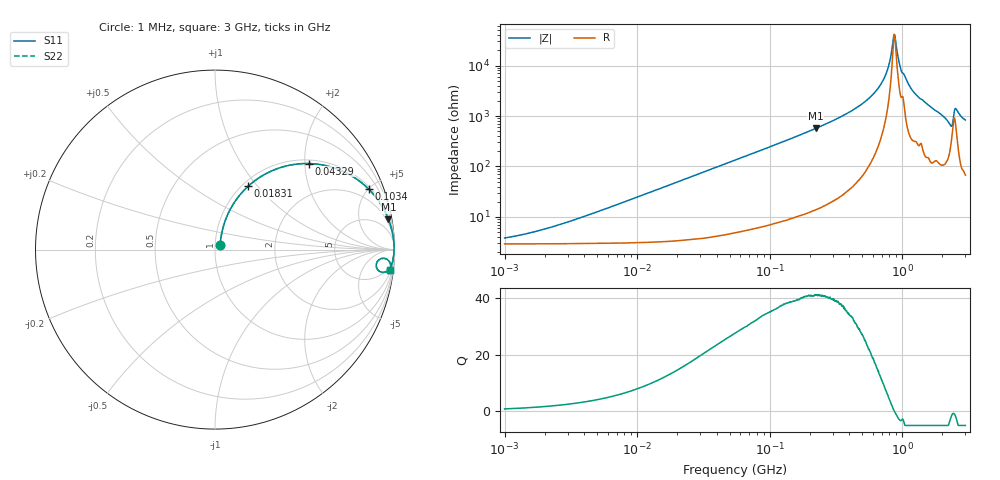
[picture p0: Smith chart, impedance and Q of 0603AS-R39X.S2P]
!s-Parameter Generated by FASTRON Sdn. Bhd.
!FASTRON P/N : 0603AS-R39X
!Keysight Technologies: E4991B_MY54100416_A.01.15
!Date: Tue Oct 17 16:06:11 2023
!Date created: Tue Oct 17 16:06:11 2023
!Version  : Rev01 Tue Oct 17 16:06:11 2023
!Data & Calibration Information:
!Freq	S11	S21	S12	S22
!PortZ  Port1:50+j0  Port2:50+j0
!When reading reference impedance value at option line is always used.
! Remarks : This data is being provided solely for informational purposes.
# Hz S dB R 50
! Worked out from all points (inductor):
!   1601 points, 1 MHz to 3 GHz, reference 50 ohm
!   read as one part in series: L = 390 nH near 3.618 MHz
!   highest Q = 41 at 222.4 MHz (marker M1), where L = 405 nH
!   self-resonance near 871.6 MHz
!   S11 on the Smith chart (normalised r, x): 1 MHz: 1.06, +0.05; 18.31 MHz: 1.07, +0.89; 43.29 MHz: 1.09, +2.11; 103.4 MHz: 1.14, +5.04; 3 GHz: 2, -17
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1000000  -28.61 38.9  -0.25 -1.4  -0.25 -1.4  -28.61 38.9
3804036  -20.47 67.2  -0.29 -5.2  -0.29 -5.2  -20.47 67.2
1.447069e7  -9.76 65.9  -0.75 -18.9  -0.75 -18.9  -9.76 65.9
1.830753e7  -8.00 62.4  -1.03 -23.4  -1.03 -23.4  -8.00 62.4
4.329325e7  -2.96 42.4  -3.42 -45.3  -3.42 -45.3  -2.96 42.4
5.477226e7  -2.09 36.1  -4.58 -51.8  -4.58 -51.8  -2.09 36.1
1.034087e8  -0.72 21.4  -8.75 -67.0  -8.75 -67.0  -0.72 21.4
2.083556e8  -0.19 10.7  -14.62 -77.9  -14.62 -77.9  -0.19 10.7
2.223601e8  -0.17 10.0  -15.23 -78.6  -15.23 -78.6  -0.17 10.0
3.817355e8  -0.06 5.1  -21.01 -83.3  -21.01 -83.3  -0.06 5.1
5.500551e8  -0.03 2.7  -26.63 -84.8  -26.63 -84.8  -0.03 2.7
6.924261e8  -0.02 1.3  -32.73 -83.8  -32.73 -83.8  -0.02 1.3
7.925923e8  -0.02 0.6  -40.10 -77.5  -40.10 -77.5  -0.02 0.6
8.501091e8  -0.02 0.2  -49.21 -50.7  -49.21 -50.7  -0.02 0.2
8.760197e8  -0.02 -0.0  -52.21 7.1  -52.21 7.1  -0.02 -0.0
8.982141e8  -0.02 -0.2  -48.66 46.6  -48.66 46.6  -0.02 -0.2
9.443041e8  -0.02 -0.4  -41.73 69.3  -41.73 69.3  -0.02 -0.4
9.828732e8  -0.03 -0.7  -38.11 72.3  -38.11 72.3  -0.03 -0.7
1.243477e9  -0.04 -2.0  -29.06 81.6  -29.06 81.6  -0.04 -2.0
2.289646e9  -0.44 -7.7  -17.12 65.4  -17.12 65.4  -0.44 -7.7
2.556106e9  -0.26 -3.7  -23.01 63.7  -23.01 63.7  -0.26 -3.7
3e9  -0.14 -6.8  -18.55 78.6  -18.55 78.6  -0.14 -6.8
